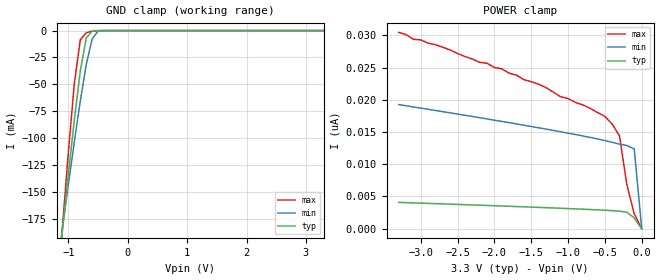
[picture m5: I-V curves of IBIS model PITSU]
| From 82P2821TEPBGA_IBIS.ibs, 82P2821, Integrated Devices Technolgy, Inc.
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|   Model PITSU
[Model]		PITSU
Model_type	Input
Polarity   Non-Inverting
Vinl = 		0.8000V
Vinh = 		2.0000V
C_comp   5.0600pF   4.7200pF   6.5800pF
[Temperature Range]	  25.0000   90.0000   -40.0000
[Voltage Range]   3.3000V   3.0000V   3.6000V
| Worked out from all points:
|   GND clamp passes 1 mA (typ) near -0.61 V on its own axis
[GND_clamp]
|Voltage	  I(typ)   I(min)   I(max)
-3.3V     -1.417A    -1.129A    -1.858A
-1.2V     -239.2mA   -225mA     -255.1mA
-1.1V     -185.7mA   -183.7mA   -182.6mA
-1V       -133.3mA   -143.1mA   -112.7mA
-900mV    -83.07mA   -103.5mA   -49.11mA
-800mV    -37.76mA   -65.72mA   -8.686mA
-700mV    -7.082mA   -31.79mA   -2.048mA
-600mV    -446.6uA   -7.71mA    -463.6uA
-500mV    -43.78uA   -564.8uA   -74.14uA
3.3V      799.4fA    13.12nA    -7.444nA
[POWER_clamp]
|Voltage	  I(typ)   I(min)   I(max)
-3.3V     4.078nA    19.26nA    30.47nA
-3.1V     4.004nA    18.9nA     29.4nA
-1.9V     3.518nA    16.65nA    24.81nA
-1.4V     3.302nA    15.66nA    22.44nA
-1.1V     3.168nA    15.04nA    20.48nA
-800mV    3.023nA    14.4nA     19.23nA
-500mV    2.862nA    13.68nA    17.44nA
-400mV    2.797nA    13.41nA    16.23nA
-300mV    2.711nA    13.12nA    14.4nA
-200mV    2.549nA    12.91nA    6.782nA
-100mV    1.673nA    12.38nA    2.323nA
0V        797fA      199pA      578.1fA
